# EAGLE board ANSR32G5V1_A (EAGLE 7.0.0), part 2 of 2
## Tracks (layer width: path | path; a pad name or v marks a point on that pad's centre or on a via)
GND  (via drill 0.5, 0.9)
  Top 0.254: 314.96,51.32 314.96,53.35 314.32,53.99 | FOR_NANO.GND@1 314.96,46.37 | 309.88,70.5 309.88,63.51 | POWER.C 340.75,25.93 X25.1
  Top 0.305: v269.37,47.51 268.61,48.27 268.61,48.82 C7.2
  Top 0.406: C1.2 C4.2 | C3.2 C2.2
  Top 1.016: X26.1 332.97,61.61 | 314.96,43.95 314.96,50.18 314.96,51.32
  Bottom 0.254: 309.88,65.42 FOR_NANO.GND
  other vias: 120.65,54.62 336.8,32.27 251.46,59.07 130.81,59.07 300.36,59.7 337.19,60.34 310.51,60.59 341,60.34 324.49,56.53 325.88,52.97 306.96,39.13
  pour Top (isolate 0.305): -2.54,32.4 -2.54,71.77 346.39,71.77 346.39,32.4
  pour Top: 346.39,20.33 335.6,20.33 335.6,32.4 346.39,32.4
  pour Bottom (isolate 0.305): -5.71,32.4 -5.71,71.77 346.07,71.77 346.07,32.4
  pour Top: 346.39,8.9 335.6,8.9 335.6,32.4 346.39,32.4
  pour Top: 346.39,9.54 335.6,9.54 335.6,32.4 346.39,32.4
I2C_SCL  (via drill 0.5, 0.6, 0.9)
  Top 0.254: v300.36,64.78 294.64,64.78 294,64.15 v294,55.26 | X26.4 319.66,53.99 319.66,54.62 318.64,55.64 316.48,55.64 316.25,55.87 RN26.3 316.23,59.52 316.23,57.8 v315.6,57.8
  Top 0.305: IC2.12 128.27,54.89 129.17,53.99 132.08,53.99 v133.35,55.26 | v248.92,55.89 IC1.12
  Top 0.406: v300.36,64.78 303.53,64.78 304.17,64.15 304.17,60.97 306.07,59.07 v307.34,59.07
  Bottom 0.254: FOR_NANO.A5 322.58,61.61 330.2,53.99 X26.4
  Bottom 0.305: v294,55.26 249.56,55.26 v248.92,55.89 247.01,55.89 245.75,54.62 220.34,54.62 219.71,55.26 135.89,55.26 135.25,55.89 133.99,55.89 v133.35,55.26
  Bottom 0.406: v307.34,59.07 314.32,59.07 v315.6,57.8
I2C_SDA  (via drill 0.5, 0.6, 0.9)
  Top 0.254: v300.36,67.32 294,67.32 292.74,66.05 v292.74,53.99 | RN26.4 317.05,59.14 v317.75,58.43 | v318.38,53.98 v318.39,53.99 | X26.3 328.93,56.53 327.66,55.26 v320.68,55.26
  Top 0.305: IC2.13 127,54.37 128.66,52.72 132.72,52.72 v134.62,54.62 | v247.65,54.62 IC1.13
  Top 0.406: v300.36,67.32 304.17,67.32 305.44,66.05 305.44,63.51 v307.34,61.61
  Bottom 0.254: v317.75,58.43 317.75,54.62 v318.39,53.99 319.66,55.26 v320.68,55.26 | FOR_NANO.A4 325.12,62.24 330.83,56.53 X26.3
  Bottom 0.305: v134.62,54.62 219.07,54.62 219.71,53.99 247.01,53.99 v247.65,54.62 292.1,54.62 v292.74,53.99
  Bottom 0.406: v307.34,61.61 314.98,61.61 RN26.4 317.05,59.14 v317.75,58.43
N$1
  Bottom 2.54: K8_B2.COM@1 193.04,74.94 | 193.04,74.94 K8_B2.COM@2 | X8.2 193.06,74.96 193.04,74.94
N$2
  Top 2.54: K8_B2.NC 190.5,87.64 187.96,90.18 187.96,93.31 X8.3
N$3
  Top 2.54: K8_B2.NO 195.58,87.64 198.12,90.18 198.12,93.31 X8.1
N$4
  Top 2.54: K7_B2.NO 210.82,88.28 213.36,90.82 213.36,93.31 X7.1
N$5
  Top 2.54: K6_B2.NO 226.06,87.64 228.6,90.18 228.6,93.31 X6.1
N$6
  Top 2.54: K7_B2.NC 205.74,87.64 203.2,90.18 203.2,93.31 X7.3
N$7
  Bottom 2.54: K7_B2.COM@1 208.28,74.94 | 208.28,74.94 K7_B2.COM@2 | X7.2 208.3,74.96 208.28,74.94
N$8
  Top 2.54: K6_B2.NC 220.98,87.64 218.44,90.18 218.44,93.31 X6.3
N$9
  Top 0.254: POWER.A 332.98,27.43 332.61,27.06 331.34,27.06 RNB1.3
  Top 0.406: 331.3,27.19 RNB1.3
N$10
  Top 2.54: K4_B2.NO 280.04,87.64 282.57,90.18 282.57,93.31 X4.1
N$11
  Top 2.54: K4_B2.NC 274.95,87.64 272.42,90.18 272.42,93.31 X4.3
N$12
  Bottom 2.54: K4_B2.COM@1 277.5,74.94 | 277.5,74.94 K4_B2.COM@2 | X4.2 277.52,74.96 277.5,74.94
N$13
  Top 0.813: 307.98,42.68 IC7.8 316.42,42.68 H1.2 | 307.98,42.68 306.2,42.68 305.44,41.92 305.44,37.38 304.93,36.87 304.93,35.46 D1.C 304.78,35.32 302.77,35.32 301.88,36.21 294.64,36.21 293.75,37.1 CD1.2 | 307.95,42.71 307.98,42.68
N$14
  Bottom 2.54: K6_B2.COM@1 223.52,74.94 | 223.52,74.94 K6_B2.COM@2 | X6.2 223.54,74.96 223.52,74.94
N$15
  Top 0.813: CD1.1 296.06,43.68 297.18,42.56 302.01,42.56 302.13,42.68 IC7.1
N$33
  Top 2.54: K5_B2.NC 236.22,87.64 233.68,90.18 233.68,93.31 X5.3
N$34
  Bottom 2.54: K5_B2.COM@2 238.76,74.94 | 238.76,74.94 K5_B2.COM@1 | X5.2 238.78,74.96 238.76,74.94
N$35
  Top 2.54: K5_B2.NO 241.3,87.64 243.84,90.18 243.84,93.31 X5.1
N$36
  Top 2.54: K3_B2.NO 295.27,87.64 297.81,90.18 297.81,93.31 X3.1
N$37
  Top 2.54: K3_B2.NC 290.19,87.64 287.65,90.18 287.65,93.31 X3.3
N$38
  Bottom 2.54: K3_B2.COM@1 292.74,74.94 | 292.74,74.94 K3_B2.COM@2 | X3.2 292.76,74.96 292.74,74.94
N$39
  Top 2.54: K2_B2.NO 310.51,87.64 313.06,90.18 313.06,93.31 X2.1
N$40
  Top 2.54: K2_B2.NC 305.44,87.64 302.89,90.18 302.89,93.31 X2.3
N$41
  Bottom 2.286: K2_B2.COM@1 307.98,74.94 K2_B2.COM@2
  Bottom 2.54: X2.2 308,74.96 307.98,74.94
N$42
  Top 2.54: K1_B2.NO 325.75,87.64 328.3,90.18 328.3,93.31 X1.1
N$43
  Top 2.54: K1_B2.NC 320.68,87.64 318.13,90.18 318.13,93.31 X1.3
N$44
  Bottom 2.54: K1_B2.COM@1 323.21,74.94 | 323.21,74.94 K1_B2.COM@2 | X1.2 323.24,74.96 323.21,74.94
N$78
  Bottom 2.54: K1_B4.COM@1 154.31,74.94 | 154.31,74.94 K1_B4.COM@2 | X9.2 154.33,74.96 154.31,74.94
N$79
  Top 2.54: K1_B4.NC 151.76,87.64 149.22,90.18 149.22,93.31 X9.3
N$80
  Top 2.54: K1_B4.NO 156.84,87.64 159.38,90.18 159.38,93.31 X9.1
N$81
  Top 2.54: K2_B4.NO 141.6,87.64 144.15,90.18 144.15,93.31 X10.1
N$82
  Top 2.54: K3_B4.NO 126.36,87.64 128.91,90.18 128.91,93.31 X11.1
N$83
  Top 2.54: K2_B4.NC 136.53,87.64 133.99,90.18 133.99,93.31 X10.3
N$84
  Bottom 2.54: K2_B4.COM@1 139.06,74.94 | 139.06,74.94 K2_B4.COM@2 | X10.2 139.09,74.96 139.06,74.94
N$85
  Top 2.54: K3_B4.NC 121.28,87.64 118.75,90.18 118.75,93.31 X11.3
N$86
  Bottom 2.54: K3_B4.COM@1 123.83,74.94 | 123.83,74.94 K3_B4.COM@2 | X11.2 123.85,74.96 123.83,74.94
N$87
  Top 2.54: K4_B4.NC 106.05,87.64 103.5,90.18 103.5,93.31 X12.3
N$88
  Bottom 2.54: K4_B4.COM@1 107.95,74.94 | 107.95,74.94 K4_B4.COM@2 | X12.2 108.61,75.6 107.95,74.94
N$89
  Top 2.54: K4_B4.NO 111.12,87.64 113.67,90.18 113.67,93.31 X12.1
N$90
  Top 2.54: K5_B4.NO 72.39,87.64 74.93,90.18 74.93,93.31 X13.1
N$91
  Top 2.54: K5_B4.NC 67.31,87.64 64.77,90.18 64.77,93.31 X13.3
N$92
  Bottom 2.54: K5_B4.COM@1 69.85,74.94 | 69.85,74.94 K5_B4.COM@2 | X13.2 69.87,74.96 69.85,74.94
N$93
  Top 2.54: K6_B4.NO 57.15,87.64 59.69,90.18 59.69,93.31 X14.1
N$94
  Top 2.54: K6_B4.NC 52.07,87.64 49.53,90.18 49.53,93.31 X14.3
N$95
  Bottom 2.54: K6_B4.COM@1 54.61,74.94 | 54.61,74.94 K6_B4.COM@2 | X14.2 54.63,74.96 54.61,74.94
N$96
  Top 2.54: K7_B4.NO 41.91,87.64 44.45,90.18 44.45,93.31 X15.1
N$97
  Top 2.54: K7_B4.NC 36.83,87.64 34.29,90.18 34.29,93.31 X15.3
N$98
  Bottom 2.54: K7_B4.COM@1 40.01,74.94 | 40.01,74.94 K7_B4.COM@2 | X15.2 39.39,75.56 40.01,74.94
N$99
  Top 2.54: K8_B4.NO 26.67,87.64 29.21,90.18 29.21,93.31 X16.1
N$100
  Top 2.54: K8_B4.NC 21.59,87.64 19.05,90.18 19.05,93.31 X16.3
N$101
  Bottom 2.54: K8_B4.COM@1 24.13,74.94 | 24.13,74.94 K8_B4.COM@2 | X16.2 24.15,74.96 24.13,74.94
N$179
  Bottom 2.54: K8_B3.COM@2 23.5,30.49 | 23.5,30.49 K8_B3.COM@1 | X17.2 23.47,30.47 23.5,30.49
N$180
  Top 2.54: K8_B3.NC 26.04,17.79 28.57,15.25 28.57,12.12 X17.3
N$181
  Top 2.54: K8_B3.NO 20.95,17.79 18.41,15.25 18.41,12.12 X17.1
N$182
  Top 2.54: K7_B3.NO 36.2,17.79 33.66,15.25 33.66,12.12 X18.1
N$183
  Top 2.54: K6_B3.NO 51.44,17.79 48.9,15.25 48.9,12.12 X19.1
N$184
  Top 2.54: K7_B3.NC 41.27,17.79 43.81,15.25 43.81,12.12 X18.3
N$185
  Bottom 2.54: K7_B3.COM@2 38.73,30.49 | 38.73,30.49 K7_B3.COM@1 | X18.2 38.71,30.47 38.73,30.49
N$186
  Top 2.54: K6_B3.NC 56.52,17.79 59.05,15.25 59.05,12.12 X19.3
N$187
  Bottom 2.54: K6_B3.COM@1 54.61,30.49 | 54.61,30.49 K6_B3.COM@2 | X19.2 53.95,29.84 54.61,30.49
N$188
  Top 2.54: K5_B3.NC 71.75,17.79 74.3,15.25 74.3,12.12 X20.3
N$189
  Bottom 2.54: K5_B3.COM@1 69.22,30.49 | 69.22,30.49 K5_B3.COM@2 | X20.2 69.19,30.47 69.22,30.49
N$190
  Top 2.54: K5_B3.NO 66.67,17.79 64.14,15.25 64.14,12.12 X20.1
N$191
  Top 2.54: K4_B3.NO 105.41,17.79 102.87,15.25 102.87,12.12 X21.1
N$192
  Top 2.54: K4_B3.NC 110.49,17.79 113.03,15.25 113.03,12.12 X21.3
N$193
  Bottom 2.54: K4_B3.COM@2 107.95,30.49 | 107.95,30.49 K4_B3.COM@1 | X21.2 107.93,30.47 107.95,30.49
N$194
  Top 2.54: K3_B3.NO 120.65,17.79 118.11,15.25 118.11,12.12 X22.1
N$195
  Top 2.54: K3_B3.NC 125.73,17.79 128.27,15.25 128.27,12.12 X22.3
N$196
  Bottom 2.54: K3_B3.COM@2 123.19,30.49 | 123.19,30.49 K3_B3.COM@1 | X22.2 123.17,30.47 123.19,30.49
N$197
  Top 2.54: K2_B3.NO 135.89,17.79 133.35,15.25 133.35,12.12 X23.1
N$198
  Top 2.54: K2_B3.NC 140.97,17.79 143.51,15.25 143.51,12.12 X23.3
N$199
  Bottom 2.54: K2_B3.COM@2 137.79,30.49 | 137.79,30.49 K2_B3.COM@1 | X23.2 138.41,29.88 137.79,30.49
N$200
  Top 2.54: K1_B3.NO 151.13,17.79 148.59,15.25 148.59,12.12 X24.1
N$201
  Top 2.54: K1_B3.NC 156.21,17.79 158.75,15.25 158.75,12.12 X24.3
N$202
  Bottom 2.54: K1_B3.COM@1 153.67,30.49 | 153.67,30.49 K1_B3.COM@2 | X24.2 153.65,30.47 153.67,30.49
N$203
  Bottom 2.54: K8_B1.COM@2 192.41,30.49 | 192.41,30.49 K8_B1.COM@1 | X251.2 192.38,30.47 192.41,30.49
N$204
  Top 2.54: K8_B1.NC 194.94,17.79 197.49,15.25 197.49,12.12 X251.3
N$205
  Top 2.54: K8_B1.NO 189.87,17.79 187.32,15.25 187.32,12.12 X251.1
N$206
  Top 2.54: K7_B1.NO 205.1,17.79 202.56,15.25 202.56,12.12 X261.1
N$207
  Top 2.54: K6_B1.NO 220.34,17.79 217.81,15.25 217.81,12.12 X271.1
N$208
  Top 2.54: K7_B1.NC 210.19,17.79 212.72,15.25 212.72,12.12 X261.3
N$209
  Bottom 2.54: K7_B1.COM@1 207.65,30.49 | 207.65,30.49 K7_B1.COM@2 | X261.2 207.62,30.47 207.65,30.49
N$210
  Top 2.54: K6_B1.NC 225.43,17.79 227.97,15.25 227.97,12.12 X271.3
N$211
  Bottom 2.54: K6_B1.COM@1 222.88,30.49 | 222.88,30.49 K6_B1.COM@2 | X271.2 222.86,30.47 222.88,30.49
N$212
  Top 2.54: K5_B1.NC 240.66,17.79 243.21,15.25 243.21,12.12 X281.3
N$213
  Bottom 2.54: K5_B1.COM@1 238.12,30.49 | 238.12,30.49 K5_B1.COM@2 | X281.2 238.1,30.47 238.12,30.49
N$214
  Top 2.54: K5_B1.NO 235.59,17.79 233.04,15.25 233.04,12.12 X281.1
N$215
  Top 2.54: K4_B1.NO 274.32,17.79 271.78,15.25 271.78,12.12 X291.1
N$216
  Top 2.54: K4_B1.NC 279.4,17.79 281.94,15.25 281.94,12.12 X291.3
N$217
  Bottom 2.54: K4_B1.COM@2 276.86,30.49 | 276.86,30.49 K4_B1.COM@1 | X291.2 276.84,30.47 276.86,30.49
N$218
  Top 2.54: K3_B1.NO 289.56,17.79 287.02,15.25 287.02,12.12 X301.1
N$219
  Top 2.54: K3_B1.NC 294.64,17.79 297.18,15.25 297.18,12.12 X301.3
N$220
  Bottom 2.54: K3_B1.COM@2 292.1,30.49 | 292.1,30.49 K3_B1.COM@1 | X301.2 292.08,30.47 292.1,30.49
N$221
  Top 2.54: K2_B1.NO 304.8,17.79 302.26,15.25 302.26,12.12 X311.1
N$222
  Top 2.54: K2_B1.NC 309.88,17.79 312.42,15.25 312.42,12.12 X311.3
N$223
  Bottom 2.54: K2_B1.COM@1 307.34,30.49 | 307.34,30.49 K2_B1.COM@2 | X311.2 307.32,30.47 307.34,30.49
N$224
  Top 2.54: K1_B1.NO 320.04,17.79 317.5,15.25 317.5,12.12 X3211.1
N$225
  Top 2.54: K1_B1.NC 325.12,17.79 327.66,15.25 327.66,12.12 X3211.3
N$226
  Bottom 2.54: K1_B1.COM@1 322.58,30.49 | 322.58,30.49 K1_B1.COM@2 | X3211.2 322.56,30.47 322.58,30.49
N$405  (via drill 0.5)
  Top 0.229: IC1.21 254,47.32 253.37,46.68 240.03,46.68 239.4,47.32 IC3.1
  Top 0.254: 254,47.32 v254,49.67 | v268.22,46.88 268.86,46.24 270.92,46.24
  Top 0.305: 270.92,46.24 270.98,46.24 RN19.5
  Bottom 0.229: v254,49.67 254,49.54 254.63,50.18 267.59,50.18 268.22,49.54 v268.22,46.88
N$406  (via drill 0.5)
  Top 0.229: IC1.25 v259.09,46.62 259.08,44.78 258.44,44.14 234.95,44.14 234.31,44.78 IC3.5 | v264.8,42.88 268.29,42.88 268.61,42.56 270.91,42.56 RN18.5
  Bottom 0.229: v259.09,46.62 259.08,47.79 259.44,48.15 264.39,48.15 264.8,47.74 v264.8,42.88
N$407  (via drill 0.5)
  Top 0.229: IC1.26 v260.35,46.62 260.35,44.46 259.4,43.51 233.68,43.51 233.04,44.14 IC3.6 | v265.75,41.92 268.29,41.92 268.61,41.6 270.9,41.6 RN18.6
  Bottom 0.229: v260.35,46.62 260.35,47.51 260.48,47.64 263.65,47.64 263.78,47.51 263.78,42.18 264.03,41.92 v265.75,41.92
N$408  (via drill 0.6)
  Top 0.305: IC2.16 v127,51.45 | v247.65,50.18 IC1.16 | RN17.6 290.43,58.67 | 290.43,58.67 290.83,59.07 290.83,66.05 290.19,66.69 U$13.A1 | 290.43,58.67 290.6,58.67 291.46,57.8 v291.46,50.81
  Bottom 0.305: v127,51.45 128.27,52.72 135.89,52.72 136.53,53.35 217.81,53.35 218.44,52.72 244.47,52.72 247.01,50.18 v247.65,50.18 248.28,50.81 v291.46,50.81
N$409  (via drill 0.5)
  Top 0.229: IC1.22 255.27,46.68 254.63,46.05 238.76,46.05 238.12,46.68 IC3.2
  Top 0.254: 255.27,46.68 v255.27,46.62 | v267.21,46.11 267.97,46.11 268.61,45.48 270.96,45.48 RN19.6
  Bottom 0.229: v255.27,46.62 255.27,49.29 255.65,49.67 266.7,49.67 267.21,49.16 v267.21,46.11
N$410  (via drill 0.5)
  Top 0.229: IC1.23 256.54,46.05 255.91,45.42 237.49,45.42 236.85,46.05 IC3.3
  Top 0.254: 256.54,46.05 v256.54,46.62 | v266.32,45.1 267.84,45.1 268.22,44.72 270.96,44.72 RN19.7
  Bottom 0.229: v256.54,46.62 256.54,48.91 256.79,49.16 265.94,49.16 266.32,48.78 v266.32,45.1
  Bottom 0.254: 266.57,44.97 v266.32,45.1
N$411  (via drill 0.5)
  Top 0.229: IC1.24 257.81,45.42 257.18,44.78 236.22,44.78 235.59,45.42 IC3.4
  Top 0.254: 257.81,45.42 v257.81,46.62 | v265.94,43.83 270.91,43.83 RN19.8
  Bottom 0.229: v257.81,46.62 257.81,48.15 258.32,48.65 264.67,48.65 265.43,47.89 265.43,44.34 v265.94,43.83
N$416  (via drill 0.6)
  Top 0.203: 238.12,55.89 238.44,56.21 244.16,56.21 245.11,57.16 245.11,59.38 245.75,60.02 262.25,60.02 262.89,60.66 v262.89,65.42
  Top 0.229: v262.89,65.42 262.89,66.31 262.13,67.07 262.13,67.85 RN21.8
  Top 0.406: v262.89,59.07 IC1.1 | IC4.8 238.12,55.89
  Bottom 0.406: v262.89,65.42 v262.89,59.07
N$417  (via drill 0.6)
  Top 0.203: IC4.7 236.85,56.21 237.36,56.72 243.65,56.72 244.47,57.54 244.47,60.02 245.11,60.66 260.99,60.66 261.62,61.29 v261.62,65.42
  Top 0.229: v261.62,65.42 261.62,66.43 261.24,66.81 261.24,67.9 RN21.7
  Top 0.406: v261.62,59.07 IC1.2
  Bottom 0.406: v261.62,65.42 v261.62,59.07
N$418  (via drill 0.6)
  Top 0.203: IC4.6 235.59,56.53 236.28,57.23 242.89,57.23 243.84,58.18 243.84,60.66 244.47,61.29 259.71,61.29 260.35,61.93 v260.35,65.42
  Top 0.229: v260.35,65.42 260.35,66.94 260.48,67.07 260.48,67.9 RN21.6
  Top 0.406: v260.35,59.07 IC1.3
  Bottom 0.406: v260.35,65.42 v260.35,59.07
N$419  (via drill 0.6)
  Top 0.203: IC4.5 234.31,56.53 235.52,57.73 242.25,57.73 243.21,58.69 243.21,61.29 243.84,61.93 258.44,61.93 259.08,62.56 v259.08,65.42
  Top 0.229: v259.08,65.42 259.08,66.56 259.59,67.07 259.59,67.85 RN21.5
  Top 0.406: v259.08,59.07 IC1.4
  Bottom 0.406: v259.08,59.07 v259.08,65.42
N$420  (via drill 0.6)
  Top 0.203: IC4.4 233.04,56.53 234.76,58.24 241.74,58.24 242.57,59.07 242.57,61.93 243.21,62.56 257.18,62.56 257.81,63.19 v257.81,65.42
  Top 0.229: v257.81,65.42 257.81,66.18 257.18,66.81 257.18,67.85 RN20.8
  Top 0.406: v257.81,59.07 IC1.5
  Bottom 0.406: v257.81,65.42 v257.81,59.07
N$421  (via drill 0.6)
  Top 0.203: IC4.3 231.78,56.53 234,58.75 241.24,58.75 241.94,59.45 241.94,62.56 242.57,63.19 255.91,63.19 256.54,63.83 v256.54,65.42
  Top 0.229: v256.54,65.42 256.54,66.56 256.29,66.81 256.29,67.9 RN20.7
  Top 0.406: v256.54,59.07 IC1.6
  Bottom 0.406: v256.54,65.42 v256.54,59.07
N$422  (via drill 0.6)
  Top 0.203: IC4.2 230.5,56.53 233.24,59.26 240.6,59.26 241.3,59.96 241.3,63.19 241.94,63.83 254.82,63.83 255.27,64.28 v255.27,65.42
  Top 0.229: IC1.7 255.27,57.16 | v255.27,65.42 255.27,66.43 255.52,66.69 255.52,67.9 RN20.6
  Top 0.406: 255.27,65.05 v255.27,65.42 | v255.27,59.07 IC1.7
  Bottom 0.406: v255.27,65.42 v255.27,59.07
N$423  (via drill 0.6)
  Top 0.203: IC4.1 229.24,56.53 232.6,59.89 240.09,59.89 240.66,60.46 240.66,63.76 241.38,64.47 253.55,64.47 254,64.91 v254,65.42
  Top 0.229: v254,65.42 254,66.43 254.63,67.07 254.63,67.85 RN20.5
  Top 0.406: v254,59.07 IC1.8
  Bottom 0.406: v254,59.07 v254,65.42
N$424  (via drill 0.5)
  Top 0.229: IC2.21 v133.35,49.35 133.35,47.26 132.96,46.88 120.02,46.88 119.38,47.51 IC5.1 | v148.59,43.83 150.26,43.83 RN22.5
  Bottom 0.229: v133.35,49.35 133.35,50.81 133.99,51.45 147.96,51.45 148.59,50.81 v148.59,43.83
N$425  (via drill 0.5)
  Top 0.229: IC5.2 118.11,47 118.75,46.37 134.62,46.37 v134.62,46.56 IC2.22 | RN22.6 147.4,42.96 v147.32,42.88
  Bottom 0.229: v147.32,42.88 147.32,50.18 146.69,50.81 135.25,50.81 134.62,50.18 v134.62,46.56
N$426  (via drill 0.5)
  Top 0.229: IC5.3 116.84,46.37 117.47,45.73 135.25,45.73 135.89,46.37 v135.89,46.56 IC2.23 | RN22.7 148.19,42.16 147.96,41.92 v146.05,41.92
  Bottom 0.229: v146.05,41.92 146.05,49.54 145.41,50.18 136.53,50.18 135.89,49.54 v135.89,46.56
N$427  (via drill 0.5)
  Top 0.229: IC5.4 115.57,45.73 116.2,45.1 136.53,45.1 137.16,45.73 v137.16,46.56 IC2.24 | RN22.8 148.34,41.36 147.96,40.97 145.1,40.97 v144.46,41.6
  Bottom 0.229: v144.46,41.6 144.46,48.83 143.75,49.54 137.79,49.54 137.16,48.91 v137.16,46.56
N$428  (via drill 0.5)
  Top 0.229: IC5.5 114.3,45.1 114.94,44.46 137.79,44.46 138.43,45.1 v138.43,46.56 IC2.25 | RN23.5 148.34,39.95 v148.27,40.02
  Bottom 0.229: v148.27,40.02 144.46,40.02 143.51,40.97 143.51,48.27 142.88,48.91 139.06,48.91 138.43,48.27 v138.43,46.56
N$429  (via drill 0.5)
  Top 0.229: IC5.6 113.03,44.46 113.67,43.83 139.06,43.83 139.7,44.46 v139.7,46.56 IC2.26 | RN23.6 147.4,39.15 v147.32,39.07
  Bottom 0.229: v147.32,39.07 144.15,39.07 142.56,40.65 142.56,47.56 141.85,48.27 140.03,48.27 IC2.26 v139.7,46.56
N$430  (via drill 0.5)
  Top 0.229: IC5.7 111.76,43.83 112.39,43.19 140.34,43.19 140.97,43.83 v140.97,46.56 IC2.27 | RN23.7 148.19,38.35 147.96,38.11 v146.05,38.11
  Bottom 0.229: v146.05,38.11 142.88,38.11 140.97,40.02 v140.97,46.56
N$431
  Top 0.229: IC2.28 142.24,43.19 | 142.24,43.19 141.6,42.56 111.12,42.56 110.49,43.19 IC5.8 | RN23.8 148.34,37.55 147.96,37.16 142.56,37.16 142.24,37.48 142.24,43.19
N$432  (via drill 0.6)
  Top 0.203: IC6.8 118.11,53 118.39,52.72 121.36,52.72 121.54,52.9 121.54,55.71 121.72,55.89 122.27,55.89 124.46,58.08 124.46,59.07 125.73,60.34 141.6,60.34 142.24,60.97 v142.24,65.42 | v142.24,59.07 IC2.1
  Top 0.229: v142.24,65.42 142.24,66.37 141.6,67 141.6,67.72 RN25.8
  Bottom 0.203: v142.24,65.42 v142.24,59.07
N$433  (via drill 0.6)
  Top 0.203: IC6.7 116.84,55.89 117.35,56.4 121.79,56.4 123.83,58.43 123.83,59.7 125.09,60.97 140.34,60.97 140.97,61.61 v140.97,65.42 | v140.97,59.07 IC2.2
  Top 0.229: v140.97,65.42 140.97,66.69 140.65,67 140.65,67.71 RN25.7
  Bottom 0.203: v140.97,65.42 v140.97,59.07
N$434  (via drill 0.6)
  Top 0.203: IC6.6 115.57,55.89 116.59,56.91 121.03,56.91 123.19,59.07 123.19,60.34 124.46,61.61 139.06,61.61 139.7,62.24 v139.7,65.42 | v139.7,59.07 IC2.3
  Top 0.229: v139.7,65.42 139.7,66.69 140.02,67 140.02,67.71 RN25.6
  Bottom 0.203: v139.7,65.42 v139.7,59.07
N$435  (via drill 0.6)
  Top 0.203: IC6.5 114.3,56.53 115.19,57.42 120.27,57.42 122.56,59.7 122.56,60.97 123.83,62.24 137.79,62.24 138.43,62.88 v138.43,65.42 | v138.43,59.07 IC2.4
  Top 0.229: v138.43,65.42 138.43,66.37 139.06,67 139.06,67.72 RN25.5
  Bottom 0.203: v138.43,65.42 v138.43,59.07
N$436  (via drill 0.6)
  Top 0.203: IC6.4 113.03,56.53 114.43,57.92 119.51,57.92 121.92,60.34 121.92,61.61 123.19,62.88 136.53,62.88 137.16,63.51 v137.16,65.42 | v137.16,59.07 IC2.5
  Top 0.229: v137.16,65.42 137.16,66.37 136.53,67 136.53,67.72 RN24.8
  Bottom 0.203: v137.16,65.42 v137.16,59.07
N$437  (via drill 0.6)
  Top 0.203: IC6.3 111.76,56.53 113.67,58.43 118.75,58.43 121.28,60.97 121.28,62.24 122.56,63.51 135.25,63.51 135.89,64.15 v135.89,65.42 | v135.89,59.07 IC2.6
  Top 0.229: v135.89,65.42 135.89,66.69 135.57,67 135.57,67.71 RN24.7
  Bottom 0.203: v135.89,65.42 v135.89,59.07
N$438  (via drill 0.6)
  Top 0.203: IC6.2 110.49,56.53 112.78,58.81 117.86,58.81 120.65,61.61 120.65,62.88 121.92,64.15 133.99,64.15 134.62,64.78 v134.62,65.42 | v134.62,59.07 IC2.7
  Top 0.229: v134.62,65.42 134.62,66.69 134.94,67 134.94,67.71 RN24.6
  Bottom 0.203: v134.62,65.42 v134.62,59.07
N$439  (via drill 0.6)
  Top 0.203: IC6.1 109.22,56.53 111.89,59.19 116.59,59.19 120.02,62.62 120.02,63.51 121.28,64.78 132.72,64.78 v133.35,65.42 | v133.35,59.07 IC2.8
  Top 0.229: v133.35,65.42 133.35,66.37 133.99,67 133.99,67.72 RN24.5
  Bottom 0.203: v133.35,65.42 v133.35,59.07
N$440
  Top 0.406: RN2.7 79.14,58.67 78.11,59.7 59.58,59.7 R30.C
N$441
  Top 0.406: RN5.1 209.62,60.27 208.91,60.97 182.76,60.97 R16.C
N$442
  Top 0.406: RN8.7 RN7.2
N$443
  Top 0.406: RN7.3 RN8.6
N$444
  Top 0.406: RN8.5 RN7.4
N$445
  Top 0.406: RN5.2 209.15,59.47 208.28,60.34 185.94,60.34 R15.C
N$446
  Top 0.406: RN4.3 77.87,54.86 75.56,57.16 72.28,57.16 R26.C
N$447
  Top 0.406: RN5.4 208.21,57.87 207.01,59.07 192.29,59.07 R13.C
N$448
  Top 0.406: RN5.5 RN6.4
N$449
  Top 0.406: RN7.1 RN8.8
N$450
  Top 0.406: RN8.1 208.35,56.46 206.38,58.43 195.47,58.43 R12.C
N$451
  Top 0.406: RN5.6 RN6.3
N$452
  Top 0.406: RN8.2 207.88,55.66 205.74,57.8 198.64,57.8 R11.C
N$453
  Top 0.406: RN6.2 RN5.7
N$454
  Top 0.406: RN5.8 RN6.1
N$455
  Top 0.406: RN3.4 RN4.5
N$456
  Top 0.406: RN2.5 80.08,60.27 79.38,60.97 53.23,60.97 R32.C
N$458
  Top 0.406: RN5.3 208.68,58.67 207.65,59.7 189.12,59.7 R14.C
N$459
  Top 0.406: RN8.3 207.41,54.86 205.1,57.16 201.81,57.16 R10.C
N$460
  Top 0.406: RN2.8 78.67,57.87 77.47,59.07 62.75,59.07 R29.C
N$461
  Top 0.406: RN4.1 78.81,56.46 76.83,58.43 65.92,58.43 R28.C
N$462
  Top 0.406: RN4.2 78.34,55.66 76.2,57.8 69.1,57.8 R27.C
N$463
  Top 0.406: RN12.4 RN11.5
N$464
  Top 0.305: R25.C 75.05,55.89
  Top 0.406: RN4.4 77.4,54.06 75.56,55.89 75.05,55.89
N$465
  Top 0.406: RN2.1 RN1.8
N$466
  Top 0.406: RN2.2 RN1.7
N$467
  Top 0.406: RN2.3 RN1.6
N$468
  Top 0.406: RN2.4 RN1.5
N$469
  Top 0.406: RN2.6 79.61,59.47 78.74,60.34 56.4,60.34 R31.C
N$470
  Top 0.406: RN8.4 206.94,54.06 205.1,55.89 204.59,55.89 R9.C
N$473
  Top 0.406: RN12.5 206.94,51.38 205.1,49.54 204.59,49.54 R1.C
N$474
  Top 0.406: RN11.6 RN12.3
N$475
  Top 0.406: RN12.6 207.41,50.58 205.1,48.27 201.81,48.27 R2.C
N$476
  Top 0.406: RN12.7 207.88,49.78 205.74,47.64 198.64,47.64 R3.C
N$477
  Top 0.406: RN9.4 RN10.5
N$478
  Top 0.406: RN10.6 RN9.3
N$479
  Top 0.406: RN9.2 RN10.7
N$480
  Top 0.406: RN10.8 RN9.1
N$481
  Top 0.406: RN12.2 RN11.7
N$482
  Top 0.406: RN10.1 208.21,47.57 207.01,46.37 192.29,46.37 R5.C
N$483
  Top 0.406: RN12.8 208.35,48.98 206.38,47 195.47,47 R4.C
N$484
  Top 0.406: RN10.3 209.15,45.97 208.28,45.1 185.94,45.1 R7.C
N$485
  Top 0.406: RN10.4 209.62,45.17 208.91,44.46 182.76,44.46 R8.C
N$486
  Top 0.406: RN10.2 208.68,46.77 207.65,45.73 189.12,45.73 R6.C
N$487
  Top 0.406: RN14.3 78.97,49.78 76.83,47.64 69.1,47.64 R19.C
N$488
  Top 0.406: RN14.2 78.5,50.58 76.2,48.27 72.28,48.27 R18.C
N$489
  Top 0.406: RN14.1 78.03,51.38 76.2,49.54 75.05,49.54 R17.C
N$490
  Top 0.406: RN16.4 80.72,45.17 80.01,44.46 53.23,44.46 R24.C
N$491
  Top 0.406: RN15.3 RN16.6
N$492
  Top 0.406: RN15.2 RN16.7
N$493
  Top 0.406: RN15.1 88.19,47.57 88.27,47.64 83.42,47.64 RN16.8
N$494
  Top 0.406: RN14.4 79.44,48.98 77.47,47 65.92,47 R20.C
N$495
  Top 0.406: RN16.3 80.25,45.97 79.38,45.1 56.4,45.1 R23.C
N$496
  Top 0.406: RN16.2 79.78,46.77 78.74,45.73 59.58,45.73 R22.C
N$497
  Top 0.406: RN16.1 79.31,47.57 78.11,46.37 62.75,46.37 R21.C
N$498  (via drill 0.6)
  Top 0.305: IC2.17 v128.27,50.18 | v244.47,50.18 244.47,51.45 245.11,52.08 v247.65,52.08 248.28,52.08 248.92,51.45 IC1.17 | U$13.B1 287.02,62.88 287.02,57.8 287.09,57.87 RN17.5 289.81,57.87 290.51,57.16 v290.51,52.08
  Bottom 0.305: v128.27,50.18 130.18,52.08 136.53,52.08 137.16,52.72 216.85,52.72 217.81,52.08 243.84,52.08 244.47,51.45 v244.47,50.18 | v247.65,52.08 v290.51,52.08
N$500
  Top 0.406: RN11.8 RN12.1
N$501
  Top 0.406: RN13.4 RN14.5
N$502
  Top 0.406: RN14.6 RN13.3
N$503
  Top 0.406: RN13.2 RN14.7
N$504
  Top 0.406: RN14.8 RN13.1
N$505
  Top 0.406: RN4.6 RN3.3
N$506
  Top 0.406: RN4.7 RN3.2
N$507
  Top 0.406: RN4.8 RN3.1
N$514
  Top 0.406: RN15.4 RN16.5
N$525  (via drill 0.5)
  Top 0.229: IC3.7 231.78,43.51 232.41,42.88 260.67,42.88 261.62,43.83 v261.62,46.62 IC1.27 | v266.7,40.97 270.43,40.97 RN18.7
  Bottom 0.229: v266.7,40.97 261.94,40.97 261.62,41.29 v261.62,46.62
N$526
  Top 0.229: IC1.28 262.89,42.88 | 262.89,42.88 262.25,42.24 231.14,42.24 230.5,42.88 IC3.8 | 262.89,42.88 262.89,40.65 263.52,40.02 270.91,40.02 RN18.8
OC_R1_A  (via drill 0.6)
  Top 0.406: IC3.18 v239.4,38.81 239.4,34.94 240.03,34.3 300.99,34.3 301.62,33.67 301.62,25.41 302.26,24.78 319.4,24.78 320.04,24.14 K1_B1.C1 | RN11.4 227.26,51.38 v227.46,51.19
  Bottom 0.406: v227.46,51.19 239.01,51.19 239.4,50.81 v239.4,38.81
OC_R1_B
  Top 0.203: RN7.5 226.13,54.06 232.73,60.66 237.17,60.66 238.12,61.61 IC4.11
  Top 0.406: IC4.11 238.12,69.23 238.76,69.86 249.56,69.86 250.19,70.5 297.81,70.5 300.1,72.91 322.45,72.91 323.21,73.67 323.21,81.93 323.85,82.56 K1_B2.C1
OC_R1_C  (via drill 0.6)
  Top 0.406: RN13.8 106.61,51.38 v106.68,51.45 | IC5.18 v119.38,38.75 119.38,36.21 120.65,34.94 148.59,34.94 149.22,34.3 149.22,23.51 149.86,22.87 K1_B3.C1
  Bottom 0.406: v106.68,51.45 118.11,51.45 119.38,50.18 v119.38,38.75
OC_R1_D
  Top 0.203: RN3.5 105.48,54.06 111.12,59.7 115.57,59.7 118.11,62.24 IC6.11
  Top 0.406: IC6.11 118.11,69.86 118.75,70.5 153.67,70.5 154.31,71.13 154.31,81.93 154.94,82.56 K1_B4.C1
OC_R2_A  (via drill 0.6)
  Top 0.406: RN11.3 225.66,50.58 v226.06,50.18 | IC3.17 v238.12,38.81 238.17,38.77 238.17,34.33 238.85,33.67 300.36,33.67 300.99,33.03 300.99,23.51 301.62,22.87 K2_B1.C1
  Bottom 0.406: v226.06,50.18 236.85,50.18 238.12,48.91 v238.12,38.81
OC_R2_B
  Top 0.203: IC4.12 236.85,62.24 235.9,61.29 232.73,61.29 226.29,54.86 RN7.6
  Top 0.406: IC4.12 236.85,69.86 237.49,70.5 248.92,70.5 249.56,71.13 297.18,71.13 299.72,73.67 307.34,73.67 307.98,74.31 307.98,81.93 308.61,82.56 K2_B2.C1
OC_R2_C  (via drill 0.6)
  Top 0.406: RN13.7 105.01,50.58 v105.41,50.18 | IC5.17 v118.11,38.75 118.11,34.94 119.38,33.67 133.35,33.67 133.99,33.03 133.99,23.51 134.62,22.87 K2_B3.C1
  Bottom 0.406: v105.41,50.18 115.57,50.18 118.11,47.64 v118.11,38.75
OC_R2_D
  Top 0.203: RN3.6 105.01,54.86 110.49,60.34 114.3,60.34 116.84,62.88 IC6.12
  Top 0.406: IC6.12 116.84,70.82 117.47,71.45 138.75,71.45 139.06,71.77 139.06,81.93 139.7,82.56 K2_B4.C1
OC_R3_A  (via drill 0.6)
  Top 0.406: RN11.2 223.92,49.78 v224.79,48.91 | IC3.16 v236.85,38.81 236.85,33.67 237.49,33.03 287.02,33.03 287.65,32.4 287.65,23.51 288.29,22.87 K3_B1.C1
  Bottom 0.406: v224.79,48.91 235.59,48.91 236.85,47.64 v236.85,38.81
OC_R3_B
  Top 0.203: RN7.7 226.46,55.66 232.73,61.93 235.27,61.93 235.59,62.24 IC4.13
  Top 0.406: IC4.13 235.59,70.5 236.22,71.13 248.28,71.13 248.92,71.77 292.1,71.77 292.74,72.4 292.74,81.93 293.37,82.56 K3_B2.C1
OC_R3_C  (via drill 0.6)
  Top 0.406: RN13.6 103.27,49.78 v104.14,48.91 | IC5.16 v116.84,38.75 116.84,34.3 118.75,32.4 118.75,23.51 119.38,22.87 K3_B3.C1
  Bottom 0.406: v104.14,48.91 114.3,48.91 116.84,46.37 v116.84,38.75
OC_R3_D
  Top 0.203: RN3.7 104.54,55.66 109.73,60.85 112.9,60.85 115.57,63.51 IC6.13
  Top 0.406: IC6.13 115.57,71.13 116.84,72.4 123.19,72.4 123.83,73.04 123.83,81.93 124.46,82.56 K3_B4.C1
OC_R4_A  (via drill 0.6)
  Top 0.406: RN11.1 222.18,48.98 v223.52,47.64 | IC3.15 v235.59,38.81 235.59,33.67 236.85,32.4 271.78,32.4 272.42,31.76 272.42,23.51 273.05,22.87 K4_B1.C1
  Bottom 0.406: v223.52,47.64 234.31,47.64 235.59,46.37 v235.59,38.81
OC_R4_B
  Top 0.203: RN7.8 226.62,56.46 232.73,62.56 234,62.56 234.31,62.88 IC4.14
  Top 0.406: IC4.14 234.31,71.13 234.95,71.77 247.65,71.77 248.6,72.72 277.18,72.72 277.5,73.04 277.5,81.93 278.13,82.56 K4_B2.C1
OC_R4_C  (via drill 0.6)
  Top 0.406: RN13.5 101.53,48.98 v102.87,47.64 | IC5.15 v115.57,38.75 115.57,33.67 114.94,33.03 109.86,33.03 109.22,33.03 108.58,33.03 107.95,32.4 107.95,23.51 107.31,22.87 K4_B3.C1
  Bottom 0.406: v102.87,47.64 113.03,47.64 115.57,45.1 v115.57,38.75
OC_R4_D
  Top 0.203: IC6.14 114.3,63.13 112.52,61.35 109.47,61.35 104.65,56.53 89.77,56.53 RN3.8
  Top 0.406: IC6.14 114.3,70.5 113.03,71.77 113.03,81.93 112.39,82.56 K4_B4.C1
OC_R5_A  (via drill 0.6)
  Top 0.406: RN9.8 221.05,47.57 222.25,46.37 v227.33,46.37 | IC3.14 v234.31,38.81 234.31,33.67 233.68,33.03 233.68,23.51 234.31,22.87 K5_B1.C1
  Bottom 0.406: v227.33,46.37 233.04,46.37 234.31,45.1 v234.31,38.81
OC_R5_B
  Top 0.203: IC4.15 233.04,63.51 232.73,63.19 232.41,63.19 227.08,57.87 RN6.5
  Top 0.406: IC4.15 233.04,71.77 233.68,72.4 242.57,72.4 243.21,73.04 243.21,81.93 242.57,82.56 K5_B2.C1
OC_R5_C  (via drill 0.6)
  Top 0.406: IC5.14 v114.3,38.75 114.3,34.94 113.67,34.3 69.85,34.3 69.22,33.67 69.22,23.51 68.58,22.87 K5_B3.C1 | RN15.8 101.03,47.57 102.23,46.37 v106.68,46.37
  Bottom 0.406: v106.68,46.37 112.39,46.37 114.3,44.46 v114.3,38.75
OC_R5_D
  Top 0.203: IC6.15 113.03,63 112.01,61.99 109.09,61.99 105.03,57.92 89.76,57.92 RN1.1
  Top 0.406: IC6.15 113.03,69.23 110.49,71.77 74.93,71.77 74.3,72.4 74.3,81.93 73.66,82.56 K5_B4.C1
OC_R6_A  (via drill 0.6)
  Top 0.406: RN9.7 220.58,46.77 222.25,45.1 v226.06,45.1 | IC3.13 v233.04,38.81 233.04,34.94 232.41,34.3 223.52,34.3 222.88,33.67 222.88,23.51 222.25,22.87 K6_B1.C1
  Bottom 0.406: v226.06,45.1 231.78,45.1 233.04,43.83 v233.04,38.81
OC_R6_B
  Top 0.203: RN6.6 226.93,58.67 231.78,63.51 IC4.16
  Top 0.406: IC4.16 231.78,71.13 230.5,72.4 228.6,72.4 227.97,73.04 227.97,81.93 227.33,82.56 K6_B2.C1
OC_R6_C  (via drill 0.6)
  Top 0.406: IC5.13 v113.03,38.75 113.03,36.21 112.39,35.57 55.24,35.57 53.98,34.3 53.98,23.51 53.34,22.87 K6_B3.C1 | RN15.7 100.56,46.77 102.23,45.1 v105.41,45.1
  Bottom 0.406: v105.41,45.1 111.76,45.1 113.03,43.83 v113.03,38.75
OC_R6_D
  Top 0.203: IC6.16 111.76,63 111.25,62.5 108.71,62.5 105.03,58.81 89.85,58.81 RN1.2
  Top 0.406: IC6.16 111.76,68.59 109.86,70.5 59.69,70.5 59.05,71.13 59.05,81.93 58.42,82.56 K6_B4.C1
OC_R7_A  (via drill 0.6)
  Top 0.406: RN9.6 220.11,45.97 222.25,43.83 v224.79,43.83 | IC3.12 v231.78,38.81 231.78,36.21 231.14,35.57 208.28,35.57 207.65,34.94 207.65,23.51 207.01,22.87 K7_B1.C1
  Bottom 0.406: v224.79,43.83 230.5,43.83 231.78,42.56 v231.78,38.81
OC_R7_B
  Top 0.203: RN6.7 226.78,59.47 230.5,63.19 IC4.17
  Top 0.406: IC4.17 230.5,70.5 229.87,71.13 213.36,71.13 212.72,71.77 212.72,81.93 212.09,82.56 K7_B2.C1
OC_R7_C  (via drill 0.6)
  Top 0.406: v111.76,38.75 IC5.12 111.76,37.61 110.87,36.72 40.39,36.72 39.24,36.72 38.73,36.21 38.73,23.51 38.1,22.87 K7_B3.C1 | RN15.6 100.09,45.97 102.23,43.83 v104.14,43.83
  Bottom 0.406: v104.14,43.83 110.49,43.83 111.76,42.56 v111.76,38.75
OC_R7_D
  Top 0.203: IC6.17 110.49,63.39 110.11,63 108.58,63 105.03,59.45 89.72,59.45 RN1.3
  Top 0.406: IC6.17 110.49,67.96 109.22,69.23 44.45,69.23 43.81,69.86 43.81,81.93 43.18,82.56 K7_B4.C1
OC_R8_A  (via drill 0.6)
  Top 0.406: RN9.5 219.64,45.17 222.25,42.56 v223.52,42.56 | IC3.11 v230.5,38.81 230.5,37.48 229.87,36.84 193.04,36.84 192.41,36.21 192.41,23.51 191.77,22.87 K8_B1.C1
  Bottom 0.406: v223.52,42.56 229.24,42.56 230.5,41.29 v230.5,38.81
OC_R8_B
  Top 0.203: RN6.8 226.62,60.27 229.24,62.88 IC4.18
  Top 0.406: IC4.18 229.24,69.86 228.6,70.5 198.12,70.5 197.49,71.13 197.49,81.93 196.85,82.56 K8_B2.C1
OC_R8_C  (via drill 0.6)
  Top 0.406: v110.49,38.75 IC5.11 110.49,41.92 109.86,42.56 107.95,42.56 107.31,41.92 107.31,38.75 106.68,38.11 24.13,38.11 23.5,37.48 23.5,23.51 22.86,22.87 K8_B3.C1 | RN15.5 99.62,45.17 102.23,42.56 v102.87,42.56
  Bottom 0.406: v102.87,42.56 109.22,42.56 110.49,41.29 v110.49,38.75
OC_R8_D
  Top 0.203: RN1.4 104.96,60.27 107.57,62.88 107.57,63.21 108.97,64.6 IC6.18
  Top 0.406: IC6.18 109.22,66.69 107.95,67.96 29.84,67.96 28.57,69.23 28.57,81.93 27.94,82.56 K8_B4.C1
REG_5V  (via drill 0.5, 0.6, 0.9)
  Top 0.254: 285.75,67.32 285.75,67 U$13.A2 | RN26.6 RN26.5 317.12,61.21 317.12,61.73 316.74,62.12 v316.74,62.5 | 329.61,27.19 328.8,27.19 328.3,26.68 328.3,23.51 329.18,22.62 v340.36,22.62
  Top 0.305: IC2.15 v125.73,53.99 126.36,53.99 129.54,50.81 129.54,47.64 | 250.19,53.99 251.46,55.26 252.09,55.26 252.73,55.89 | IC2.9 132.08,56.53 v130.81,55.26 | IC1.18 v250.19,53.35 | IC1.9 252.73,55.89 | 252.73,55.89 253.37,55.26 263.84,55.26 264.16,55.26 265.43,56.53 270.51,56.53 | 270.51,56.53 281.31,56.53 284.48,59.7 285.75,59.7 285.99,59.47 | 286.22,63.68 U$13.B2 U$13.A2 | C1.1 270.6,56.44 270.51,56.53 | 329.61,27.19 RNB1.6
  Top 0.406: C2.1 C3.1 | C4.1 C1.1 | IC2.18 129.54,50.81 130.18,51.45 144.55,51.45 | C8.1 144.55,51.45 | 144.55,51.45 C5.1 144.55,45.96 144.78,45.73 149.54,45.73 149.86,46.05 149.86,46.37 | C6.1 C7.1 265.2,54.22 264.16,55.26 | 149.86,47.64 149.86,47.72 | 149.86,47.72 C3.1 | C3.1 149.86,47.96 149.86,47.72
  Top 0.61: v316.74,62.5 318.52,62.5 321.94,59.07 X26.2
  Top 0.813: H1.1 311.63,36.69 v311.15,36.21 | IC7.4 302.39,38.87 | 302.39,38.87 v302.26,38.75 | 302.39,38.87 299.32,38.87 C10.1
  Top 1.016: 154.94,45.73 150.18,45.73 149.86,46.05 | 149.86,46.37 149.86,47.64 | C24.+ 156.21,47 154.94,45.73 | C28.+ 156.21,44.46 154.94,45.73 | C1.1 270.6,48.18 271.4,47.38 275.46,47.38 276.23,46.62 276.23,46.37 | 276.23,46.37 C25.+ | C27.+ 284.48,45.1 283.21,46.37 276.23,46.37 | C26.+ 269.24,56.85
  Top 1.27: 285.75,67 U$13.B2 285.75,60.02 284.16,60.02 280.99,56.85 269.24,56.85 265.43,56.85 263.84,55.26 253.05,55.26 252.73,55.58 251.78,55.58 250.19,53.99 v250.19,53.35 | H1.1 320.14,35.42 v320.68,35.83
  Bottom 0.254: v340.36,22.62 341.25,21.73 342.9,21.73 344.17,23 344.17,43.19 344.81,43.83 344.81,58.43 344.17,59.07 v339.47,59.07
  Bottom 0.305: v250.19,53.35 219.07,53.35 218.44,53.99 135.89,53.99 135.25,53.35 133.99,53.35 133.35,53.99 v125.73,53.99 125.73,54.62 126.36,55.26 v130.81,55.26
  Bottom 0.61: FOR_NANO.5V 314.96,64.27 | 314.96,64.27 v316.74,62.5 | 314.96,64.27 314.96,64.15 314.32,63.51 302.89,63.51 301.62,62.24
  Bottom 0.813: v311.15,36.21 302.26,36.21 v302.26,38.75 300.99,40.02 300.99,50.81 302.26,52.08 302.26,61.61 301.62,62.24 v300.36,62.24
  Bottom 1.016: v339.47,59.07 X26.2 | v300.36,62.24 287.02,62.24 285.75,63.51 U$13.B2
REG_12V  (via drill 0.5)
  Top 0.813: BRA2.+ 327.02,40.02 325.12,37.48 317.5,37.48 313.69,41.29 311.4,41.29 v307.21,41.41 IC7.7 | C9.1 299.21,51.32 300.36,50.18 301.62,50.18 302.26,49.54 v302.26,44.46
  Bottom 0.813: v302.26,44.46 302.26,42.56 303.4,41.41 v307.21,41.41
UNREG_12V  (via drill 0.6)
  Top 0.305: 204.47,52.72 R1.A
  Top 0.406: IC5.10 v109.22,38.75 | IC6.10 119.38,66.05 v120.02,66.69 | IC4.10 v239.4,62.56 | R8.A 177.8,52.72 | R15.A 181.61,52.72 | R6.A 185.42,52.72 | 189.23,52.72 R13.A | R4.A 193.04,52.72 | R3.A 196.85,52.72 | R2.A 200.66,52.72 | R16.A 177.8,52.72 | 177.8,52.72 181.61,52.72 | R7.A 181.61,52.72 | 181.61,52.72 185.42,52.72 | R14.A 185.42,52.72 | 185.42,52.72 189.23,52.72 | R5.A 189.23,52.72 | 189.23,52.72 193.04,52.72 | R12.A 193.04,52.72 | 193.04,52.72 196.85,52.72 | R11.A 196.85,52.72 | 196.85,52.72 200.66,52.72 | R10.A 200.66,52.72 | R24.A 48.26,52.72 | R31.A 52.07,52.72 | R30.A 55.88,52.72 | R29.A 59.69,52.72 | R28.A 63.5,52.72 | v67.31,52.72 R19.A | 71.12,52.72 R18.A | R25.A 74.93,52.72 | 74.93,52.72 R17.A | R32.A 48.26,52.72 | 48.26,52.72 52.07,52.72 | R23.A 52.07,52.72 | 52.07,52.72 55.88,52.72 | R22.A 55.88,52.72 | 55.88,52.72 59.69,52.72 | R21.A 59.69,52.72 | 59.69,52.72 63.5,52.72 | R20.A 63.5,52.72 | 63.5,52.72 v67.31,52.72 | v67.31,52.72 71.12,52.72 | R26.A 71.12,52.72 | 71.12,52.72 74.93,52.72 | R9.A 204.47,52.72 | 204.47,50.81 204.47,52.72 | 204.47,52.72 202.25,52.72 | 200.66,52.72 202.25,52.72 | 202.25,52.72 v202.25,49.54 | IC3.10 229.24,39.38 v229.2,38.81 | R27.A v67.31,52.72
  Top 2.54: BRA2.~@2 BRA2.~@1 331.42,34.94 U$14.TIP 332.13,36.27 332.13,33.33 336.23,29.22 341.94,29.22 X25.2
  Bottom 0.406: v239.4,62.56 239.4,71.13 238.76,71.77 | v202.25,49.54 202.25,33.67 | 229.3,33.99 229.62,33.67 | v67.31,52.72 67.31,33.67
  Bottom 0.813: v109.22,38.75 109.22,33.67
  Bottom 1.016: 229.3,33.99 229.2,33.99 v229.2,38.81 | 220.34,71.13 219.71,71.77 | 31.11,71.13 31.75,71.77 | C22.+ 171.45,34.3 170.81,33.67 | C23.+ 219.07,71.77 | C21.+ 147.96,71.77 | C20.+ 12.7,43.19 | C19.+ 12.7,66.69 | K8_B4.C2 19.68,82.56 19.05,81.93 19.05,71.77 | K7_B4.C2 34.92,82.56 34.29,81.93 34.29,72.4 33.66,71.77 | K6_B4.C2 50.16,82.56 49.53,81.93 49.53,71.77 | K5_B4.C2 65.41,82.56 64.77,81.93 64.77,72.4 64.14,71.77 | K4_B4.C2 104.14,82.56 103.5,81.93 103.5,71.77 | K3_B4.C2 119.38,82.56 118.75,81.93 118.75,71.77 | K2_B4.C2 134.62,82.56 133.99,81.93 133.99,72.4 134.62,71.77 | K1_B4.C2 149.86,82.56 149.22,81.93 149.22,72.4 149.86,71.77 | K8_B2.C2 188.59,82.56 187.96,81.93 187.96,71.77 | K7_B2.C2 203.84,82.56 203.2,81.93 203.2,72.4 203.84,72.4 204.47,71.77 | K6_B2.C2 219.07,82.56 218.44,81.93 218.44,71.77 | K5_B2.C2 234.31,82.56 233.68,81.93 233.68,72.4 233.04,71.77 | K4_B2.C2 273.05,82.56 272.42,81.93 272.42,71.77 | K3_B2.C2 288.29,82.56 287.65,81.93 287.65,71.77 288.29,71.77 289.56,73.04 302.89,73.04 | K2_B2.C2 303.53,82.56 302.89,81.93 302.89,73.04 | K1_B1.C2 327.02,22.87 327.66,23.51 327.66,33.67 | K2_B1.C2 311.79,22.87 312.42,23.51 312.42,33.03 313.06,33.67 | K3_B1.C2 296.55,22.87 297.18,23.51 297.18,33.03 297.81,33.67 | K4_B1.C2 281.31,22.87 281.94,23.51 281.94,33.03 282.57,33.67 | K5_B1.C2 242.57,22.87 243.21,23.51 243.21,33.67 | K6_B1.C2 227.33,22.87 227.97,23.51 227.97,33.67 | K7_B1.C2 212.09,22.87 212.72,23.51 212.72,33.67 | K8_B1.C2 196.85,22.87 197.49,23.51 197.49,33.03 196.85,33.67 | K1_B3.C2 158.75,22.87 159.38,23.51 159.38,33.67 | K2_B3.C2 142.88,22.87 143.51,23.51 143.51,33.67
  Bottom 1.016: K3_B3.C2 127.64,22.87 128.27,23.51 128.27,33.03 128.91,33.67 | K4_B3.C2 112.39,22.87 113.03,23.51 113.03,33.67 | K5_B3.C2 73.66,22.87 74.3,23.51 74.3,33.03 74.93,33.67 | K6_B3.C2 58.42,22.87 59.05,23.51 59.05,33.67 | K7_B3.C2 43.18,22.87 43.81,23.51 43.81,33.67 | K8_B3.C2 27.94,22.87 28.57,23.51 28.57,33.67 | K1_B2.C2 318.77,82.56 318.13,81.93 318.13,74.31 316.87,73.04 302.89,73.04
  Bottom 1.27: v120.02,66.69 120.02,71.77
  Bottom 2.54: 332.74,33.67 332.36,33.29 336.13,29.52 | 332.74,33.67 327.66,33.67 313.06,33.67 297.81,33.67 282.57,33.67 243.21,33.67 229.62,33.67 227.97,33.67 212.72,33.67 202.25,33.67 196.85,33.67 170.81,33.67 159.38,33.67 143.51,33.67 128.91,33.67 113.03,33.67 109.22,33.67 74.93,33.67 67.31,33.67 59.05,33.67 43.81,33.67 28.57,33.67 12.7,33.67 12.7,43.19 12.7,66.69 12.7,71.77 19.05,71.77 31.75,71.77 33.66,71.77 49.53,71.77 64.14,71.77 103.5,71.77 118.75,71.77 120.02,71.77 134.62,71.77 147.96,71.77 149.86,71.77 187.96,71.77 204.47,71.77 218.44,71.77 219.07,71.77 219.71,71.77 233.04,71.77 238.76,71.77 272.42,71.77 287.65,71.77 | 332.74,33.67 332.13,33.33 332.13,36.27 U$14.TIP

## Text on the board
tNames: NC | COM | NO | NC | COM | NO | NC | COM | NO | NC | COM | NO | NC | COM | NO | NC | COM | NO | NC | COM | NO | NC | COM | NO | NC | COM | NO | NC | COM | NO | NC | COM | NO | NC | COM | NO | NC | COM | NO | NC | COM | NO | NC | COM | NO | NC | COM | NO | 8 | 5 | 4 | 1 | 8 | 5 | 4 | 1 | NC | COM | NO | NC | COM | NO | NC | COM | NO | NC | COM | NO | NC | COM | NO | NC | COM | NO | NC | COM | NO | NC | COM | NO | NC | COM | NO | NC | COM | NO | NC | COM | NO | NC | COM | NO | NC | COM | NO | NC | COM | NO | NC | COM | NO | NC | COM | NO | ANSR32G5V1 | Bank 4 | Bank 2 | MCP23017 | REV.A | Address: | A1 | A2 | GND | +5V | SC | SDA | SCL | 2016 ControlEverything.com | Address A0=0 | Address A0=1 | Bank 3 | Bank 1 | NO | COM | NC | NO | COM | NC | NO | COM | NC | NO | COM | NC | NO | COM | NC | NO | COM | NC | NO | COM | NC | NO | COM | NC | NO | COM | NC | NO | COM | NC | NO | COM | NC | NO | COM | NC | NO | COM | NC | NO | COM | NC | NO | COM | NC | NO | COM | NC | 8 | 5 | 4 | 1 | 8 | 5 | 4 | 1 | 12V DC / Power / Supply | 12V DC / Power / Supply | 12V DC / Power / Supply | NO | COM | NC | NO | COM | NC | NO | COM | NC | NO | COM | NC | NO | COM | NC | NO | COM | NC | NO | COM | NC | NO | COM | NC | NO | COM | NC | NO | COM | NC | NO | COM | NC | NO | COM | NC | NO | COM | NC | NO | COM | NC | NO | COM | NC | NO | COM | NC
